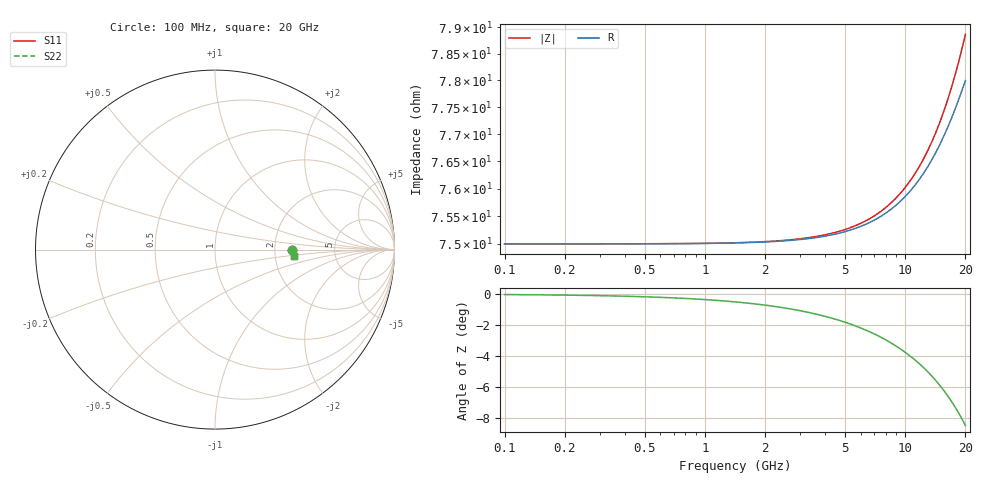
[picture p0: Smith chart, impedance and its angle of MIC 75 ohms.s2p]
! Vishay ElectroFilms Inc.
! MIC001 7500B - 75 Ohm in Series Configuration
! March 2012
# GHz S MA R 50
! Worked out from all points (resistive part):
!   233 points, 100 MHz to 20 GHz, reference 50 ohm
!   read as one part in series: R = 75 ohm at 102.3 MHz
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0.1  0.4286 -0.0  0.5714 0.0  0.5714 0.0  0.4286 -0.0
0.2436751  0.4286 -0.1  0.5714 0.0  0.5714 0.0  0.4286 -0.1
0.5937753  0.4286 -0.1  0.5714 0.1  0.5714 0.1  0.4286 -0.1
0.9375335  0.4286 -0.2  0.5714 0.1  0.5714 0.1  0.4286 -0.2
1.414214  0.4286 -0.3  0.5714 0.2  0.5714 0.2  0.4286 -0.3
1.818091  0.4287 -0.4  0.5713 0.3  0.5713 0.3  0.4287 -0.4
2.284535  0.4288 -0.5  0.5713 0.4  0.5713 0.4  0.4288 -0.5
2.805834  0.4289 -0.6  0.5712 0.4  0.5712 0.4  0.4289 -0.6
3.446086  0.429 -0.7  0.5711 0.5  0.5711 0.5  0.429 -0.7
4.430234  0.4293 -0.9  0.5708 0.7  0.5708 0.7  0.4293 -0.9
5.566843  0.4297 -1.2  0.5705 0.9  0.5705 0.9  0.4297 -1.2
6.837118  0.4302 -1.4  0.57 1.1  0.57 1.1  0.4302 -1.4
8.397251  0.4311 -1.8  0.5693 1.3  0.5693 1.3  0.4311 -1.8
9.630449  0.4319 -2.1  0.5686 1.6  0.5686 1.6  0.4319 -2.1
11.04475  0.4329 -2.4  0.5678 1.8  0.5678 1.8  0.4329 -2.4
12.38075  0.434 -2.7  0.5669 2.1  0.5669 2.1  0.434 -2.7
13.87836  0.4353 -3.1  0.5658 2.4  0.5658 2.4  0.4353 -3.1
15.20587  0.4366 -3.4  0.5648 2.6  0.5648 2.6  0.4366 -3.4
16.66035  0.4381 -3.8  0.5636 3.0  0.5636 3.0  0.4381 -3.8
18.25396  0.44 -4.2  0.5622 3.3  0.5622 3.3  0.44 -4.2
19.10705  0.441 -4.5  0.5614 3.5  0.5614 3.5  0.441 -4.5
20  0.4421 -4.8  0.5606 3.7  0.5606 3.7  0.4421 -4.8
